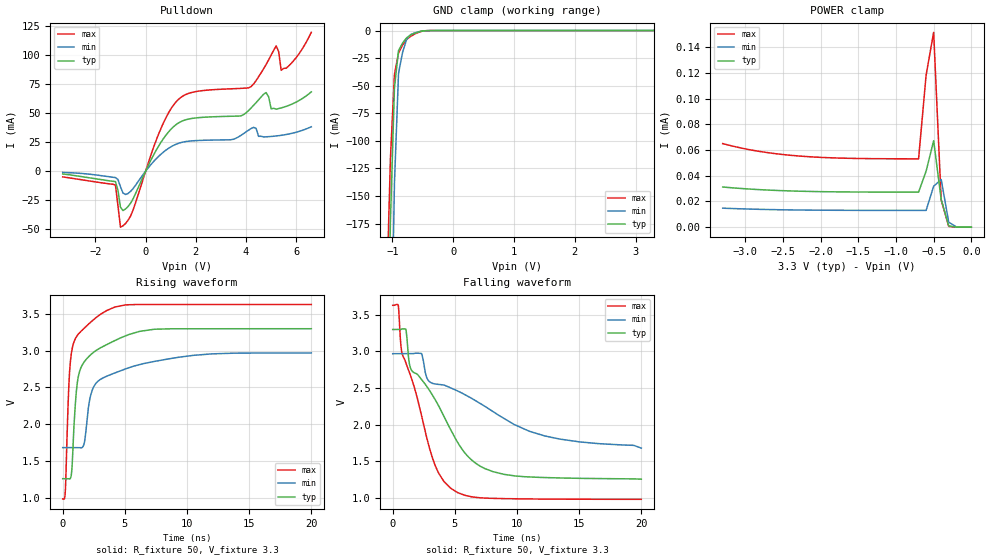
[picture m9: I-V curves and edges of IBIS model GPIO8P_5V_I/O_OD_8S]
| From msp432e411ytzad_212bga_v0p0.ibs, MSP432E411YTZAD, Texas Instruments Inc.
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|   Model Cell GPIO8P_5V_I/O_OD_8S
|GPIO8P_5V_I/O_OD_8S
[Model]   GPIO8P_5V_I/O_OD_8S
Model_type   I/O_open_drain
Polarity   Inverting
Enable   Active-Low
Vinl =  0.8
Vinh =  2
Cref =  15.0000pF
Rref =  100.0000M
Vref =  0V
Vmeas =  1.65
C_comp   7.738177p   6.063161p   9.392973p
[Model Spec]
Vinl   0.8   0.8   0.8
Vinh   2   2   2
[Temperature Range]   25   125   -40
[Voltage Range]   3.3   2.97   3.63
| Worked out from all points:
|   slope of the pulldown table from 0 to 0.495 V, typ, clamps not added: 23.8 ohm
|   GND clamp passes 1 mA (typ) near -0.55 V on its own axis
|   rising waveform, R_fixture 50, V_fixture 3.3: 20-80 % time 1.11ns typ, 2.53ns min, 573ps max; typ from 1.26 V to 3.3 V
|   falling waveform, R_fixture 50, V_fixture 3.3: 20-80 % time 4.29ns typ, 8.01ns min, 2.62ns max; typ from 3.3 V to 1.26 V
| Nom Voltages:
|   VDDC=1.2, VDD=3.3, GND=0
| Min Voltages:
|   VDDC=1.08, VDD=2.97, GND=0
| Max Voltages:
|   VDDC=1.32, VDD=3.63, GND=0
[POWER_clamp]
|   voltage   I(typ)   I(min)   I(max)
-3.3V     31.22uA    14.77uA    64.95uA
-2.8V     29.13uA    13.84uA    58.77uA
-2.3V     27.98uA    13.34uA    55.36uA
-1.7V     27.4uA     13.1uA     53.62uA
-700mV    27.24uA    13.03uA    53.12uA
-600mV    43.52uA    13.03uA    118.2uA
-500mV    67.2uA     31.8uA     151.5uA
-400mV    21.58uA    37.04uA    21.1uA
-300mV    927.4nA    3.873uA    611.4nA
-200mV    28.93nA    266.5nA    11.51nA
0V        696.9pA    10.99nA    568.3pA
[Pulldown]
|   voltage   I(typ)   I(min)   I(max)
-3.3V     -2.325mA   -1.011mA   -4.829mA
-1.2V     -8.9mA     -5.443mA   -11.78mA
-1V       -30.94mA   -13.35mA   -48.07mA
-900mV    -33.77mA   -18.67mA   -46.9mA
-500mV    -23.82mA   -14.99mA   -33.55mA
600mV     24.46mA    14.43mA    36.18mA
1.3V      41.39mA    23.95mA    61.62mA
4.2V      54.39mA    36.75mA    72.77mA
4.8V      67.66mA    29.61mA    91.8mA
5.2V      53.41mA    30.34mA    107.8mA
5.4V      54.46mA    30.89mA    86.79mA
6.6V      68.25mA    38.26mA    119.5mA
[GND_clamp]
|   voltage   I(typ)   I(min)   I(max)
-3.3V     -16.36A    -15.34A    -17.18A
-1.1V     -382.1mA   -633.4mA   -250.1mA
-1.033V   -173.3mA   -336.5mA   -116.4mA
-966.7mV  -52.02mA   -138.4mA   -39.81mA
-900mV    -18.21mA   -38.98mA   -20.34mA
-833.3mV  -11.36mA   -19.82mA   -13.17mA
-766.7mV  -6.618mA   -8.051mA   -8.134mA
-700mV    -3.983mA   -3.675mA   -5.247mA
-500mV    -328.3uA   -388.2uA   -374.5uA
-366.7mV  -15.94uA   -32.84uA   -14.83uA
3.3V      696.9pA    8.348uA    426.1pA
[Ramp]
| variable   typ   min   max
dV/dt_f   1.231019/4.291597n  0.77759801/8.0026194n  1.5950638/2.6215481n
dV/dt_r  1.2345266/3.7273164n 0.87505534/7.2485224n  1.5897027/2.2683384n
R_load = 50
[Rising Waveform]
R_fixture = 50
V_fixture = 3.3
V_fixture_min = 2.97
V_fixture_max = 3.63
|   time   V(typ)   V(min)   V(max)
0s        1.258V     1.681V     981.8mV
205ps     1.258V     1.681V     1.072V
510.2ps   1.255V     1.681V     2.587V
756ps     1.432V     1.681V     3.025V
1.007ns   2.25V      1.681V     3.162V
1.263ns   2.656V     1.681V     3.229V
1.712ns   2.845V     1.729V     3.304V
2.63ns    2.998V     2.546V     3.445V
7.35ns    3.293V     2.854V     3.63V
20.01ns   3.3V       2.97V      3.63V
[Falling Waveform]
R_fixture = 50
V_fixture = 3.3
V_fixture_min = 2.97
V_fixture_max = 3.63
|   time   V(typ)   V(min)   V(max)
0s        3.3V       2.97V      3.63V
445.7ps   3.3V       2.97V      3.633V
682.7ps   3.303V     2.97V      3.043V
1.058ns   3.303V     2.97V      2.844V
1.451ns   2.765V     2.97V      2.664V
2.33ns    2.616V     2.969V     2.12V
3.17ns    2.413V     2.567V     1.563V
4.678ns   1.93V      2.503V     1.132V
8.058ns   1.361V     2.182V     996mV
20.01ns   1.258V     1.681V     982.8mV
